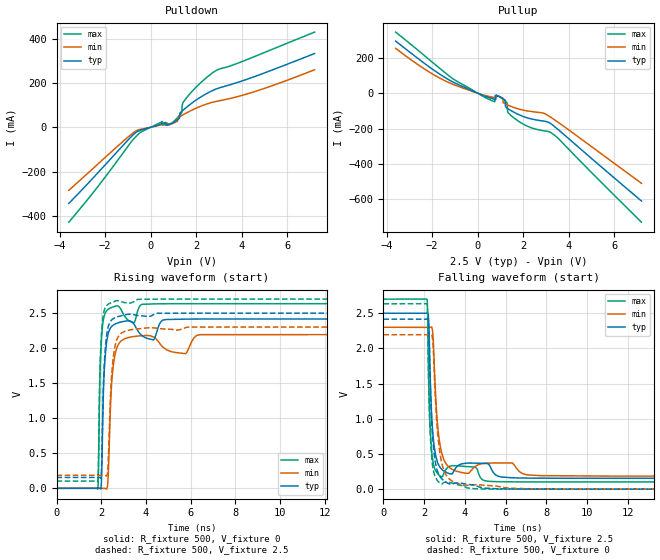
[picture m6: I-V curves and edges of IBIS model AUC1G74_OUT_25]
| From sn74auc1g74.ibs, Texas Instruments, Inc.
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[Model]   AUC1G74_OUT_25
Model_type  Output
Vref =   0
Rref =   500
Cref =   30p
Vmeas =   1.25
| variable   typ   min   max
C_comp   6.34pF   1.25pF   18.20pF
| C_pullup   6.17pF   1.25pF   15.49pF
| C_pulldown   6.51pF   2.46pF   18.20pF
[Temperature Range]   40   100   -40
| Ambient temperature   25   85   -40
[Voltage range]   2.5   2.3   2.7
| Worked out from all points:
|   slope of the pulldown table from 0 to 0.375 V, typ, clamps not added: 30.8 ohm
|   slope of the pullup table from 0 to 0.375 V, typ, clamps not added: 19.2 ohm
|   rising waveform, R_fixture 500, V_fixture 0: 20-80 % time 152ps typ, 202ps min, 118ps max; typ from 0 V to 2.42 V
|   falling waveform, R_fixture 500, V_fixture 2.5: 20-80 % time 228ps typ, 311ps min, 160ps max; typ from 2.5 V to 0.154 V
|   rising waveform, R_fixture 500, V_fixture 2.5: 20-80 % time 153ps typ, 205ps min, 118ps max; typ from 0.154 V to 2.5 V
|   falling waveform, R_fixture 500, V_fixture 0: 20-80 % time 241ps typ, 335ps min, 164ps max; typ from 2.42 V to 0 V
[Pulldown]
| AUC1G74_OUT_25
|   Voltage   I(typ)   I(min)   I(max)
-3.6V     -344.4mA   -285mA     -429.1mA
-680mV    -25.49mA   -18.73mA   -45.26mA
510mV     16.97mA    12.66mA    25.84mA
520mV     17.32mA    12.92mA    9.344mA
985mV     20.92mA    18.24mA    23.43mA
1.265V    40.56mA    47.18mA    53.79mA
1.28V     62.44mA    48.07mA    55.53mA
1.365V    72.41mA    53.05mA    65.54mA
1.395V    75.02mA    54.8mA     105.1mA
1.54V     87.47mA    63.08mA    128.4mA
2.605V    160.3mA    109.8mA    237.5mA
7.2V      333.2mA    259.7mA    430.1mA
[Pullup]
| AUC1G74_OUT_25
|   Voltage   I(typ)   I(min)   I(max)
-3.6V     294mA      252.9mA    345mA
-1.29V    77.74mA    61.54mA    101.4mA
610mV     -29.45mA   -21.35mA   -41.05mA
960mV     -19.88mA   -19.18mA   -19.53mA
1.21V     -38.96mA   -59.75mA   -44.51mA
1.225V    -74.32mA   -60.68mA   -46.11mA
1.29V     -83.38mA   -64.6mA    -53.15mA
1.335V    -87.45mA   -67.22mA   -108.8mA
1.73V     -116.5mA   -86.39mA   -152.4mA
2.885V    -157.3mA   -112.5mA   -211.7mA
3.39V     -189.2mA   -151mA     -238.4mA
7.2V      -608.9mA   -508.8mA   -728.4mA
[Ramp]
| AUC1G74_OUT_25
| variable   typ   min   max
dV/dt_r   1.46/1.52E-10   1.32/2.02E-10   1.59/1.19E-10
dV/dt_f   1.41/2.28E-10   1.27/3.12E-10   1.56/1.60E-10
R_load = 500
[Rising Waveform]
| AUC1G74_OUT_25
R_fixture =   500
C_fixture =   0
L_fixture =   0
V_fixture =   0
V_fixture_min = 0
V_fixture_max = 0
|   Time   V(typ)   V(min)   V(max)
0s        11.34nV    33.64nV    1.934nV
1.84ns    127.1uV    -5.045uV   -12.44mV
2ns       37.68mV    -14.85uV   2.073V
2.055ns   771.1mV    121.6uV    2.307V
2.12ns    1.582V     74.43uV    2.444V
2.23ns    2.057V     -9.633mV   2.529V
2.305ns   2.199V     145.1mV    2.553V
2.47ns    2.31V      1.521V     2.581V
2.67ns    2.351V     1.978V     2.603V
29.99ns   2.416V     2.195V     2.634V
[Falling Waveform]
| AUC1G74_OUT_25
R_fixture =   500
C_fixture =   0
L_fixture =   0
V_fixture =   2.5
V_fixture_min = 2.3
V_fixture_max = 2.7
|   Time   V(typ)   V(min)   V(max)
0s        2.5V       2.3V       2.7V
2.145ns   2.501V     2.3V       2.696V
2.21ns    2.456V     2.3V       1.749V
2.255ns   2.084V     2.3V       1.17V
2.365ns   1.067V     2.305V     560.4mV
2.645ns   390.7mV    961mV      228.6mV
2.87ns    280.3mV    506.8mV    175.4mV
4.085ns   370mV      224.1mV    321.3mV
5.515ns   201.3mV    372.4mV    107.5mV
29.99ns   154.5mV    185.2mV    102.7mV
[Rising Waveform]
| AUC1G74_OUT_25
R_fixture =   500
C_fixture =   0
L_fixture =   0
V_fixture =   2.5
V_fixture_min = 2.3
V_fixture_max = 2.7
|   Time   V(typ)   V(min)   V(max)
0s        154.5mV    185.2mV    102.6mV
1.84ns    154.6mV    185.2mV    90.25mV
2ns       192.7mV    185.2mV    2.148V
2.055ns   910.3mV    185.3mV    2.386V
2.125ns   1.701V     185.1mV    2.528V
2.235ns   2.171V     175.6mV    2.604V
2.305ns   2.297V     338.3mV    2.625V
2.46ns    2.401V     1.589V     2.65V
2.66ns    2.44V      2.086V     2.675V
29.99ns   2.5V       2.3V       2.7V
[Falling Waveform]
| AUC1G74_OUT_25
R_fixture =   500
C_fixture =   0
L_fixture =   0
V_fixture =   0
V_fixture_min = 0
V_fixture_max = 0
|   Time   V(typ)   V(min)   V(max)
0s        2.416V     2.195V     2.634V
2.145ns   2.417V     2.195V     2.63V
2.25ns    2.054V     2.195V     1.166V
2.365ns   994mV      2.2V       477mV
2.44ns    661.8mV    2.032V     288.5mV
2.64ns    269.2mV    879.1mV    127.3mV
2.855ns   149.8mV    384mV      73.55mV
3.5ns     87.18mV    95.63mV    74.72mV
6.34ns    2.776mV    11.7mV     511.8uV
29.99ns   24.33uV    2.255uV    12.11uV
